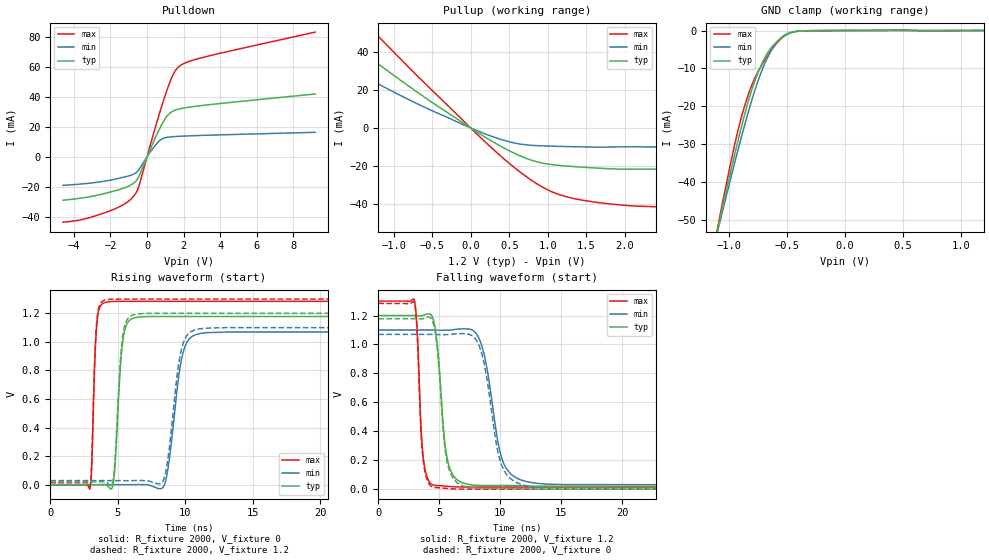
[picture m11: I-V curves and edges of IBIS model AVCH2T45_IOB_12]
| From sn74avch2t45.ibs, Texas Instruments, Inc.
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[Model]   AVCH2T45_IOB_12
Model_type  I/O
Vinl=0.385
Vinh=0.845
Enable   Active-High
Vref =   0
Rref =   2000
Cref =   15p
Vmeas =   0.6
| variable   typ   min   max
C_comp   5.41pF   4.77pF   5.94pF
| C_pullup   5.90pF   3.96pF   7.94pF
| C_pulldown   5.45pF   4.80pF   7.14pF
| C_tri-state   5.41pF   4.77pF   5.94pF
[Temperature Range]   40   100   -40
| Ambient temperature   25   85   -40
[Voltage range]   1.2   1.1   1.3
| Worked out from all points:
|   slope of the pulldown table from 0 to 0.18 V, typ, clamps not added: 34.6 ohm
|   slope of the pullup table from 0 to 0.18 V, typ, clamps not added: 38.6 ohm
|   GND clamp passes 1 mA (typ) near -0.50 V on its own axis
|   rising waveform, R_fixture 2000, V_fixture 0: 20-80 % time 434ps typ, 806ps min, 264ps max; typ from 0 V to 1.18 V
|   falling waveform, R_fixture 2000, V_fixture 1.2: 20-80 % time 678ps typ, 1.23ns min, 404ps max; typ from 1.2 V to 0.02 V
|   rising waveform, R_fixture 2000, V_fixture 1.2: 20-80 % time 428ps typ, 782ps min, 261ps max; typ from 0.02 V to 1.2 V
|   falling waveform, R_fixture 2000, V_fixture 0: 20-80 % time 676ps typ, 1.22ns min, 402ps max; typ from 1.18 V to 0 V
[GND Clamp]
| AVCH2T45_IOB_12
|   Voltage   I(typ)   I(min)   I(max)
-4.6V     -599.5mA   -548.1mA   -664.5mA
-1.095V   -51.65mA   -52.16mA   -51.03mA
-1.07V    -48.2mA    -49.03mA   -47.15mA
-940mV    -30.92mA   -33.24mA   -28.27mA
-840mV    -19.11mA   -21.95mA   -17.27mA
-775mV    -12.93mA   -15.39mA   -12.23mA
-695mV    -7.282mA   -8.82mA    -7.866mA
-615mV    -3.733mA   -4.168mA   -4.305mA
-545mV    -1.871mA   -1.692mA   -1.969mA
-465mV    -604.4uA   -486.8uA   -527.9uA
-355mV    -86uA      -70.97uA   -92.21uA
1.2V      714.8pA    1.474uA    -44.11nA
[Pulldown]
| AVCH2T45_IOB_12
|   Voltage   I(typ)   I(min)   I(max)
-4.6V     -28.79mA   -18.92mA   -43.46mA
-3.415V   -27.06mA   -17.81mA   -41.32mA
-2.035V   -23.45mA   -15.53mA   -35.96mA
-1.17V    -20.3mA    -13.14mA   -30.86mA
-680mV    -16.87mA   -11.13mA   -25.38mA
-435mV    -12.68mA   -8.327mA   -19.06mA
440mV     12.38mA    7.543mA    19.04mA
955mV     24.67mA    12.69mA    39.57mA
1.42V     30.53mA    13.49mA    54.64mA
1.79V     32.04mA    13.78mA    60.61mA
3.17V     34.51mA    14.41mA    66.63mA
9.2V      41.96mA    16.4mA     83.17mA
[Pullup]
| AVCH2T45_IOB_12
|   Voltage   I(typ)   I(min)   I(max)
-4.6V     40.24mA    7.956mA    186.3mA
-4.08V    45.4mA     8.808mA    167.8mA
-3.73V    53.62mA    9.647mA    154.2mA
-2.685V   79.31mA    16.98mA    111.4mA
-2.57V    75.87mA    21.96mA    106.5mA
-2.565V   75.72mA    49.42mA    106.3mA
-1.845V   53.66mA    37.03mA    75.82mA
-1.36V    38.76mA    26.71mA    55.3mA
575mV     -13.51mA   -7.977mA   -21.19mA
1.01V     -19.08mA   -9.527mA   -32.92mA
1.455V    -20.71mA   -9.971mA   -38.21mA
9.2V      -28.28mA   -12.48mA   -52.65mA
[Ramp]
| AVCH2T45_IOB_12
| variable   typ   min   max
dV/dt_r   0.72/4.48E-10   0.66/8.26E-10   0.79/2.79E-10
dV/dt_f   0.72/6.85E-10   0.65/1.24E-09   0.78/4.10E-10
R_load = 2000
[Rising Waveform]
| AVCH2T45_IOB_12
R_fixture =   2000
C_fixture =   0
L_fixture =   0
V_fixture =   0
V_fixture_min = 0
V_fixture_max = 0
|   Time   V(typ)   V(min)   V(max)
0s        18.14nV    102.1nV    431.7pV
2.935ns   8.853uV    929.1nV    -26.33mV
3.435ns   -98.93uV   -3.215uV   1.111V
4.025ns   1.829mV    6.876uV    1.275V
4.655ns   561.7uV    4.845uV    1.283V
5.345ns   987mV      -49.48uV   1.284V
6.175ns   1.167V     279.7uV    1.284V
8.455ns   1.178V     -1.156mV   1.284V
10.8ns    1.178V     1.052V     1.284V
40ns      1.178V     1.069V     1.284V
[Falling Waveform]
| AVCH2T45_IOB_12
R_fixture =   2000
C_fixture =   0
L_fixture =   0
V_fixture =   1.2
V_fixture_min = 1.1
V_fixture_max = 1.3
|   Time   V(typ)   V(min)   V(max)
0s        1.2V       1.1V       1.3V
2.955ns   1.2V       1.1V       1.308V
3.66ns    1.2V       1.1V       237.6mV
4.47ns    1.184V     1.1V       29.18mV
5.61ns    227.8mV    1.098V     20.18mV
6.905ns   42.79mV    1.108V     15mV
8.36ns    25.55mV    1.02V      14.48mV
10.07ns   25.81mV    227.1mV    14.45mV
11.67ns   23.55mV    64.13mV    14.45mV
40ns      20.07mV    28.67mV    14.44mV
[Rising Waveform]
| AVCH2T45_IOB_12
R_fixture =   2000
C_fixture =   0
L_fixture =   0
V_fixture =   1.2
V_fixture_min = 1.1
V_fixture_max = 1.3
|   Time   V(typ)   V(min)   V(max)
0s        20.07mV    28.66mV    14.44mV
2.93ns    20.08mV    28.66mV    -12.18mV
3.425ns   19.98mV    28.66mV    1.123V
3.99ns    22.01mV    28.67mV    1.291V
4.655ns   30.43mV    28.67mV    1.299V
5.325ns   1.012V     28.62mV    1.3V
6.135ns   1.189V     28.85mV    1.3V
8.385ns   1.2V       32.6mV     1.3V
10.7ns    1.2V       1.084V     1.3V
40ns      1.2V       1.1V       1.3V
[Falling Waveform]
| AVCH2T45_IOB_12
R_fixture =   2000
C_fixture =   0
L_fixture =   0
V_fixture =   0
V_fixture_min = 0
V_fixture_max = 0
|   Time   V(typ)   V(min)   V(max)
0s        1.178V     1.069V     1.284V
2.95ns    1.178V     1.069V     1.292V
3.655ns   1.178V     1.069V     222.8mV
4.445ns   1.163V     1.069V     15.05mV
5.59ns    209.2mV    1.068V     5.218mV
6.9ns     22.97mV    1.075V     465.9uV
8.295ns   5.68mV     984.3mV    39.76uV
9.97ns    5.777mV    200.4mV    8.781uV
11.61ns   3.267mV    35.61mV    2.863uV
40ns      403.7nV    5.655uV    185.3nV
